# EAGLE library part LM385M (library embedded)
Voltage Ref LM385M Texas Instruments
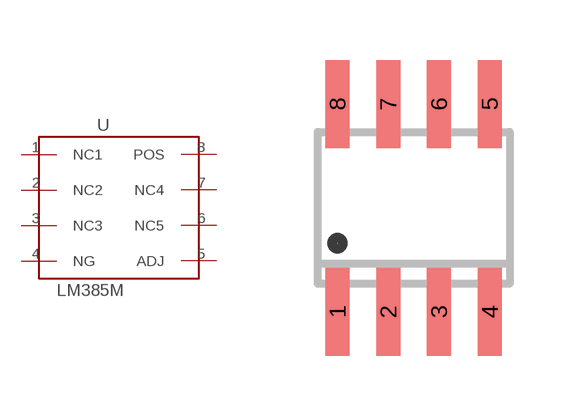
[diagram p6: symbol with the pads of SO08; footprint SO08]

Designator prefix U

## LM385M (DATASHEET: http://www.ti.com/lit/ds/symlink/lm385-adj.pdf; DESCR: Voltage References Adj MicroPwr Vtg Ref - 1.24 V to 5.3 V - SOIC-8; MF: Texas Instruments; MF_PN: LM385M/NOPB; MOUSER_NO: 926-LM385M/NOPB; PACKAGE: SOIC-8; PURCHASE: https://www.mouser.de/ProductDetail/Texas-Instruments/LM385M-NOPB?qs=QbsRYf82W3GRxYR5I5VL9w==; UNIT_PRICE: 0.83)  [SO08]
1  NC1  nc
2  NC2  nc
3  NC3  nc
4  NG
5  ADJ
6  NC5  nc
7  NC4  nc
8  POS

## Footprint SO08 (pad centres in mm)
Small Outline Package 8 NS Package M08A
smd 0.6 x 2.2: 1 -1.905,-2.6; 2 -0.635,-2.6; 3 0.635,-2.6; 4 1.905,-2.6; 5 1.905,2.6; 6 0.635,2.6; 7 -0.635,2.6; 8 -1.905,2.6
